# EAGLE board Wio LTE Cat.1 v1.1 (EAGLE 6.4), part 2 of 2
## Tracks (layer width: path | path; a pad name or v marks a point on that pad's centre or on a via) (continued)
N$49  (via drill 0.2 pad 0.41) (continued)
  VDD_3V3 0.305: v30.99,45.34 32,44.32 v33.91,44.32
N$50
  Top 0.127: U4.20 25.82,21.79 C28.1
N$51
  Bottom 0.127: U8.1 44.81,47.1 45.09,47.37 45.09,48.13 R81.1
N$52  (via drill 0.2 pad 0.41)
  Top 0.127: J11.2 8.27,40.66 v8,40.39
  Bottom 0.127: v8,40.39 7.87,40.51 R114.1 C57.1
N$53  (via drill 0.2 pad 0.41)
  Top 0.127: 17.78,6.42 v17.78,6.1 17.14,5.46 J10.3 | 17.78,6.42 D5.1 17.91,6.66 R17.1 | 17.78,6.42 17.78,6.6
  Bottom 0.127: v17.78,6.1 17.78,6.35 TP4.T
N$54  (via drill 0.2 pad 0.41)
  Top 0.127: J11.1 8.68,38.66 v8,37.97
  Bottom 0.127: R117.1 6.73,38.74 C62.1 v8,37.97
N$55  (via drill 0.2 pad 0.41)
  Top 0.127: 17.13,6.43 v17.13,6.09 16.5,5.46 J10.2 | 17.13,6.43 D3.1 17.02,6.66 R16.1 | 17.13,6.43 17.13,6.59 17.14,6.6
  Bottom 0.127: v17.13,6.09 17.13,6.37 TP3.T
N$56
  Top 0.127: R44.2 19.56,26.31 D17.-
N$57
  Bottom 0.127: U8.2 45.33,46.6 R96.1 R79.2
N$58
  Bottom 0.305: U8.3 R99.1
N$59
  Bottom 0.127: R25.2 11.81,12.19 12.95,11.05 20.32,11.05 24.13,7.24 25.53,7.24 26.29,6.48 28.51,6.48 28.89,6.1 D11.1 30.16,6.1 30.91,6.84 J2.P2B 38.59,6.84 40.64,8.89 40.64,12.06 40.01,12.7 J2.P2
  Bottom 0.152: C21.1 R25.2
N$60
  Bottom 0.127: 30.61,10.16 29.46,9.02 29.46,7.87 29.21,7.62 D10.1 28.89,7.62 28.51,8 24.64,8 21.21,11.43 13.84,11.43 13.34,11.94 R26.2 | 30.67,10.22 30.61,10.16 | 30.61,10.16 30.87,10.16 J2.P3B 37.75,10.44 38.96,11.66 J2.P3
  Bottom 0.152: C20.1 R26.2
N$61
  Bottom 0.305: C56.2 45.59,45.21 | 45.59,45.21 45.72,45.34 | 45.72,45.34 46.36,45.98 R99.2 | U8.4 45.2,45.6 45.42,45.38 | 45.42,45.38 45.59,45.21 | 45.42,45.38 45.68,45.38 45.72,45.34
N$62  (via drill 0.2 pad 0.41)
  Top 0.127: v41.53,9.27 v40.01,9.27 | v26.54,6.86 26.04,7.37 v26.04,8.64
  Bottom 0.127: v40.01,9.27 39.85,9.24 J2.P7B 30.87,9.24 29.84,8.22 29.84,7.49 29.21,6.86 D8.1 28.89,6.86 28.51,7.24 26.92,7.24 v26.54,6.86 | v41.53,9.27 41.53,5.33 38.96,2.77 J2.P7 | C19.1 14.1,12.19 14.48,11.81 21.21,11.81 24.38,8.64 v26.04,8.64
  Bottom 0.152: C19.1 R27.2 R23.2
N$63  (via drill 0.2 pad 0.41)
  Top 0.127: J12.3 7.6,28.69 v7.37,28.45
  Bottom 0.127: v7.37,28.45 7.24,28.58 C114.1 R118.1
N$64  (via drill 0.2 pad 0.41)
  Top 0.127: v7.37,27.3 8.26,27.3 8.87,26.69 J12.2
  Bottom 0.127: v7.37,27.3 7.24,27.43 R119.1 C64.1
N$65  (via drill 0.2 pad 0.41)
  Top 0.127: J12.1 8.46,24.69 8.13,25.02 v8.13,26.04
  Bottom 0.127: v8.13,26.04 7.75,26.04 7.24,26.55 R120.1 C115.1
N$66
  Top 0.127: Q9.3 35.43,4.95 R91.1
N$67  (via drill 0.25 pad 0.51)
  Top 0.127: J13.3 8.78,14.72 8.64,14.86 8.64,17.27 v8.26,17.65
  Bottom 0.127: C117.1 R121.1 v8.26,17.65
N$68
  Bottom 0.305: Q14.3 2.41,34.29 2.67,34.29 3.17,33.78 3.17,33.02 3.56,32.64 R103.1 3.56,32 Q13.1
N$69  (via drill 0.25 pad 0.51)
  Top 0.127: J13.2 8.75,12.72 8.38,13.08 8.38,15.49 v8.13,15.75
  Bottom 0.127: C116.1 7.88,15.5 v8.13,15.75 7.88,16 R122.1
N$70  (via drill 0.25 pad 0.51)
  Top 0.127: J13.1 8.46,10.72 7.87,11.3 v7.87,13.34
  Bottom 0.127: v7.87,13.34 v7.88,13.34 C126.1 R123.1
N$71
  Top 0.127: J15.3 36.43,26.69 35.81,27.3 35.81,29.59 34.54,30.86 C128.1 R129.1
N$72
  Top 0.127: U4.8 31.69,22.99 32,23.3 C42.2
N$73
  Top 0.127: J15.2 36.59,28.69 36.32,28.96 36.32,31.37 36.2,31.5 34.67,31.5 34.54,31.62 C127.1 R130.1
N$74
  Top 0.127: J15.1 37.26,30.69 36.7,31.24 36.7,32.26 36.32,32.64 34.67,32.64 34.54,32.77 C129.1 R131.1
N$75  (via drill 0.2 pad 0.41)
  Top 0.127: J16.3 42.24,12.72 v45.15,15.62
  Bottom 0.127: C131.1 45.21,15.62 v45.15,15.62 R124.1
N$76  (via drill 0.2 pad 0.41)
  Top 0.127: J16.2 43.35,14.72 v45.15,16.51
  Bottom 0.127: C130.1 v45.15,16.51 R127.1
N$77  (via drill 0.2 pad 0.41)
  Top 0.127: J16.1 44.53,16.72 45.15,17.34 v45.15,17.4
  Bottom 0.127: C132.1 v45.15,17.4 R128.1
N$78
  Top 0.127: U4.11 29.81,24.09 30.42,24.7 C26.2
N$79
  Top 0.127: U4.12 29.41,24.33 29.65,24.57 C26.1
N$80
  Top 0.127: U4.13 29.01,25.07 C27.2
N$81
  Top 0.127: U4.14 28.61,24.48 28.32,24.77 C27.1
N$82
  Bottom 0.127: Q3.3 8.51,9.27 7.24,10.54 Q2.1 5.59,10.54 5.08,11.05 5.08,12.95 R136.1
N$83
  Bottom 0.127: R135.1 C137.1 R137.2 4.44,5.21 Q3.1
N$85
  Top 0.127: U4.16 27.81,24.13 27.43,24.51 C36.1
N$87
  Top 0.127: Q6.1 31.37,33.78 R143.1 30.86,35.3 Q7.3
N$88
  Top 0.127: Q7.1 30.86,38.23 C143.1 | C143.1 R144.2 | C143.1 R142.1
N$89
  Top 0.254: U4.17 26.92,22.99 26.26,23.66 C29.1
N$90
  Top 0.203: C47.2 R53.1 | U4.29 29.41,18.21 C48.1
  Top 0.254: 29.41,18.22 C48.1 C47.2
N$93  (via drill 0.2 pad 0.41)
  Top 0.127: U4.21 26.28,21.39 v26.23,21.34
  VDD_3V3 0.127: v26.23,21.34 26.1,21.46 7.24,21.46 5.33,23.37 5.33,29.08 v5.84,29.59
  Bottom 0.127: v5.84,29.59 R42.2
N$94  (via drill 0.2 pad 0.41)
  Top 0.127: U4.22 26.45,20.99 26.29,20.83 v26.04,20.83 25.78,20.83 C44.1
  VDD_3V3 0.127: v26.04,20.83 25.65,21.21 7.11,21.21 5.08,23.24 5.08,30.48 v5.46,30.86
  Bottom 0.127: R41.2 v5.46,30.86
N$95  (via drill 0.2 pad 0.41)
  Top 0.127: U4.23 26.43,20.59 v26.16,20.32 26.04,20.32 25.91,20.19 C41.1
  VDD_3V3 0.127: v26.16,20.32 25.91,20.32 25.27,20.95 6.99,20.95 4.83,23.11 4.83,31.37 v5.08,31.62
  Bottom 0.127: v5.08,31.62 R40.2
N$96  (via drill 0.2 pad 0.41)
  Top 0.127: U4.24 26.79,20.19 v26.04,19.43 25.91,19.43 C40.1 25.53,18.92
  VDD_3V3 0.127: v26.04,19.43 24.77,20.7 6.86,20.7 4.57,22.99 4.57,32.38 v4.7,32.51
  Bottom 0.127: v4.7,32.51 R39.2
N$97
  Top 0.127: U4.32 32.41,19.59 R48.1
N$98
  Bottom 0.254: Q14.1 3.3,35.43 2.79,35.94 R102.1 R104.2 C91.1
N$99
  Top 0.127: U4.30 29.81,18.58 C46.1
N$100
  Bottom 0.305: Q15.1 3.56,19.94 R106.1 3.56,20.83 3.3,21.08 2.29,21.08 1.78,21.59 Q16.3
N$105
  Top 0.127: R91.2 34.16,3.51 D24.-
N$107
  Top 0.254: U4.19 25.69,22.19 C33.1
N$110
  Top 0.305: Q10.3 35.81,10.67 R93.1
N$111
  Top 0.127: R93.2 34.16,8.85 D25.-
N$113
  Bottom 0.305: R107.2 C93.1 R105.1 2.79,24.51 3.56,23.75 Q16.1 3.94,23.62
N$114
  Bottom 0.305: R109.2 C98.2 ANT1.D
N$115
  Bottom 0.305: R110.2 C100.2 | C100.2 25.45,52.07 L1.1 | C100.2 ANT2.D
N$118
  Bottom 0.305: L1.2 26.4,52.98 R111.1
N$120
  Top 0.127: R70.2 R71.1 36,19.65 C80.2
N$121
  Top 0.127: R72.1 R73.2 35.37,19.65 C80.1
N$123
  Top 0.127: J3.1 31.1,2.79 31.5,2.79 32.13,3.43 32.13,4.57 32.96,5.4 32.96,12.37 32.37,12.95 31.5,12.95 31.11,13.34 R82.2
N$129
  Top 0.127: 36.29,1.14 K3.4 36.58,1.43 36.58,1.91 36.57,1.91 R29.1
N$130
  Top 0.127: R30.1 7.11,5.33 7.87,6.1 9.65,6.1 10.46,5.28 K4.4
N$132
  Top 0.127: R78.2 21.59,5.78 D18.1 21.66,3.74 21.97,3.43 23.68,3.43 J3.6
N$134
  Top 0.127: J3.2 31.18,5.08 32.26,5.08 32.64,5.46 32.64,11.94 32,12.57 31.24,12.57 30.35,13.46 R75.2
NET_MODE  (via drill 0.2 pad 0.41)
  Top 0.127: R94.2 34.16,13.08 v34.04,12.95 Q10.1
  Bottom 0.127: U1.5 31.75,16.51 31.75,16 32.26,15.49 33.02,15.49 33.4,15.11 33.4,13.72 34.04,13.08 v34.04,12.95
NET_STATUS  (via drill 0.2 pad 0.41)
  Top 0.127: R92.2 34.16,7.24 Q9.1 33.4,6.99 v33.4,12.64
  Bottom 0.127: v33.4,12.64 33.4,13.21 33.02,13.59 33.02,14.99 32.77,15.24 31.24,15.24 30.35,16.13 30.35,16.61 U1.6
NRST  (via drill 0.2 pad 0.41)
  Top 0.127: 33.91,2.35 33.12,2.35 D14.- | 33.91,2.35 37.27,2.35 v38.35,3.43 | U3.7 21.7,42.05 21.34,42.42 20.57,42.42 19.81,43.18 v19.81,44.32 C23.1 | D27.1 33.91,2.35
  Top 0.305: K3.2 38.41,3.48 v38.35,3.43
  VDD_3V3 0.203: v38.35,3.43 19.18,3.43 18.54,4.06 18.54,6.1 16.89,7.75 14.1,7.75 13.34,8.51 9.02,8.51 5.97,11.56 5.97,20.45 3.68,22.73 3.68,32.89 1.91,34.67 v1.91,38.73 1.91,45.74 3.16,46.99 18.16,46.99 19.81,45.34 v19.81,44.32
  Bottom 0.305: v1.91,38.73 J4.5 | J4.5
OE
  Top 0.127: R89.1 R125.1 | R125.1 17.65,19.56 17.78,19.68 18.67,19.68 18.8,19.82 U9.10 | R125.1 R126.2
OSC32_IN
  Top 0.127: U3.3 23.7,42.12 24,42.42 25.27,42.42 25.78,42.93 C10.1 25.72,43.43 25.34,43.81 25.34,44.51 26.02,45.2 X1.1
OSC32_OUT
  Top 0.127: U3.4 23.2,42.38 23.5,42.67 24.38,42.67 24.64,42.93 C11.1 25.08,43.88 25.08,44.51 24.4,45.2 X1.2
OSC_IN
  Top 0.127: U3.5 22.7,42.64 23.37,43.31 23.37,43.76 X3.1
OSC_OUT
  Top 0.127: U3.6 22.2,42.18 21.21,43.18 21.21,43.63 X3.3
PWRKEY  (via drill 0.2 pad 0.41)
  Top 0.127: K4.2 6.88,1.38 6.1,2.16 D26.1 | 6.06,5.23 D26.1 | v6.6,18.67 7.11,18.16 7.11,14.48 6.86,14.22 6.86,12.95 5.59,11.68 5.59,5.46 5.78,5.26 D26.1
  Bottom 0.127: U1.21 9.18,25.18 8.51,24.51 6.6,24.51 6.29,24.19 6.29,21.59 7.11,20.77 R85.1 6.99,20.2 6.22,19.43 R37.2 6.1,19.18 v6.6,18.67
PWRKEY_MODULE  (via drill 0.2 pad 0.41)
  Top 0.127: v6.99,24.13 6.99,34.67 8.64,36.32 13.72,36.32 14.23,35.81 U3.24
  Bottom 0.127: v6.99,24.13 7.18,23.94 Q1.1 8,23.5 R38.2
RESET_MODULE
  Top 0.127: U3.11 19.7,34.5 16,30.8 16,27.56 16.2,27.36 U9.15
RESET_N  (via drill 0.2 pad 0.41)
  Top 0.127: U9.6 16.2,21.79 v16.26,21.84
  VDD_3V3 0.127: v16.26,21.84 16.13,21.72 13.21,21.72 v11.43,23.5
  Bottom 0.127: v11.43,23.5 11.43,23.62 11.17,23.88 U1.20
RGB_POWR  (via drill 0.2 pad 0.41)
  Top 0.127: U3.41 21.2,30.48 22.73,32 v22.73,35.81
  Bottom 0.127: R8.2 8.13,37.21 8.38,37.47 11.56,37.47 13.08,35.94 17.02,35.94 17.78,35.18 20.7,35.18 21.34,35.81 v22.73,35.81
RI_MODULE  (via drill 0.2 pad 0.41)
  Top 0.127: U9.1 12.95,24.38 v13.84,25.27
  Bottom 0.127: v13.84,25.27 15.88,25.27 16.64,26.04 16.64,27.84 18.01,29.21 20.57,29.21 24.13,32.77 26.16,32.77 26.54,33.15 26.54,34.54 26.92,34.92 36.77,34.92 37.42,35.58 U1.62
RX_LED
  Top 0.127: U3.34 17.7,28.4 18.41,27.69 18.42,27.69 R44.1
RXD_MODULE  (via drill 0.2 pad 0.41)
  Top 0.127: U9.5 15.55,21.77 16.38,22.61 v17.4,22.61
  Bottom 0.127: v17.4,22.61 17.4,24.77 17.78,25.15 35.18,25.15 36.07,26.04 36.07,27.18 36.67,27.78 U1.68
SD_CLK
  Bottom 0.127: J2.T5 37.91,15.23 38.69,16 41.4,16 41.91,16.51 D20.1 42.09,17.2 C18.1 R64.2 R60.1
SD_CMD
  Bottom 0.127: J2.T3 36.86,1.49 36.45,1.91 36.45,2.67 35.69,3.43 28.32,3.43 27.11,4.64 26.23,4.64 26.04,4.83 D22.1 25.97,5.08 C17.1 R58.1 R63.2
SD_DATA0
  Bottom 0.102: 38.92,16.51 38.86,16.51 37.47,15.11 36.32,15.11 35.81,14.6
  Bottom 0.127: R61.1 R65.2 C60.1 40.13,16.58 D19.1 38.92,16.51 | J2.T7 35.81,14.6
SD_POWR  (via drill 0.2 pad 0.41)
  Top 0.127: U3.50 24.97,32.31 24,33.27 v24,34.16
  VDD_3V3 0.127: v4.83,36.45 6.86,34.42 20.32,34.42 20.83,33.91 23.75,33.91 v24,34.16
  Bottom 0.127: v4.83,36.45 4.7,36.58 R102.2
SDIO_CK  (via drill 0.2 pad 0.41)
  Top 0.127: U3.53 27.51,33.81 27.88,33.44 v27.88,29.15
  Bottom 0.127: v27.88,29.15 27.94,29.21 35.05,29.21 36.83,30.99 40.39,30.99 41.4,29.97 42.42,29.97 43.81,28.57 43.81,20.32 R60.2
SDIO_CMD  (via drill 0.2 pad 0.41)
  Top 0.127: U3.54 25.8,34.31 v25.78,34.29
  VDD_3V3 0.127: v25.78,34.29 25.4,33.91 25.4,33.02 26.04,32.38 26.04,28.7 27.18,27.56 27.18,20.04 27.54,19.68 28.77,19.68 29.21,19.24 29.21,18.34 28.71,17.84 26.86,17.84 26.67,17.65 25.02,17.65 24.26,16.89 24.26,10.03 22.8,8.57 v22.23,8.57
  Bottom 0.127: v22.23,8.57 24.38,6.41 R58.2
SDIO_D0  (via drill 0.2 pad 0.41)
  Top 0.127: U3.39 20.2,29.16 21.04,28.32 v21.14,28.32
  Bottom 0.127: R61.2 41.4,20.07 43.05,20.07 43.56,20.57 43.56,28.44 42.28,29.72 36.58,29.72 35.24,28.38 21.21,28.38 v21.14,28.32
SDIO_D1  (via drill 0.2 pad 0.41)
  Top 0.127: U3.40 20.7,30.61 v21.21,31.11
  VDD_3V3 0.127: v23.11,11.3 23.75,11.94 23.75,17.14 24.77,18.16 26.42,18.16 26.61,18.35 28.44,18.35 28.7,18.61 28.7,18.99 28.51,19.18 27.18,19.18 26.67,19.68 26.67,24.38 21.21,29.84 v21.21,31.11
  Bottom 0.127: R57.2 v23.12,11.3 v23.11,11.3
SDIO_D2  (via drill 0.2 pad 0.41)
  Top 0.127: U3.51 25.48,32.81 v25.02,33.27
  VDD_3V3 0.127: v21.72,8.38 21.72,8.64 22.23,9.14 22.99,9.14 24,10.16 24,17.02 24.89,17.91 26.54,17.91 26.73,18.1 28.59,18.1 28.96,18.47 28.96,19.11 28.64,19.43 27.38,19.43 26.92,19.89 26.92,27.43 25.78,28.57 25.78,32.26 25.02,33.02 v25.02,33.27
  Bottom 0.127: R5.2 24.38,1.02 24.26,0.89 23.11,0.89 21.46,2.54 21.46,8.13 v21.72,8.38
SDIO_D3  (via drill 0.2 pad 0.41)
  Top 0.127: U3.52 25.82,33.31 v25.78,33.27
  VDD_3V3 0.127: v25.78,33.27 26.29,32.77 26.29,28.83 27.43,27.69 27.43,20.19 27.69,19.94 28.96,19.94 29.46,19.43 29.46,18.22 28.83,17.59 27.05,17.59 26.86,17.4 25.15,17.4 24.51,16.76 24.51,9.91 22.61,8 v22.23,8
  Bottom 0.127: R24.2 23.12,3.17 22.86,3.43 22.86,4.32 21.84,5.33 21.84,7.62 v22.23,8
SPK_L
  Top 0.203: C28.2 24.26,21.46 23.75,20.95 23.75,18.67 arc90 24,18.41 24.45,18.41 arc-90 24.7,18.16 arc-90 24.45,17.91 24,17.91 arc90 23.75,17.65 arc90 24,17.4 24.45,17.4 arc-90 24.7,17.14 arc-90 24.45,16.89 24,16.89 arc90 23.75,16.51 23.75,15.05 23.88,14.92 24.13,14.92 C88.2 C87.1 C96.1 26.73,15.05 26.8,15.11 D9.1 27.4,15.3 R83.1
SPK_R
  Top 0.203: C29.2 25.11,24.86 24.51,24.26 24.51,23.37 23.37,22.23 23.37,14.92 23.69,14.61 24,14.61 24.13,14.48 C86.2 C89.2 C97.2 26.74,14.48 D13.1 27.27,14.42 R84.1
STATUS  (via drill 0.2 pad 0.41)
  Top 0.127: v21.27,34.29 18.7,31.72 U3.36 18.7,28.79 19.18,28.32 20.45,28.32 R101.1
  Bottom 0.127: v21.27,34.29 22.04,35.05 25.02,35.05 25.78,35.81 35.89,35.81 36.96,36.88 U1.61
TX_LED
  Top 0.127: U3.35 18.2,28.66 18.8,28.07 19.94,28.07 R43.1
TXD_MODULE  (via drill 0.2 pad 0.41)
  Top 0.127: U9.4 14.9,22.14 v14.99,22.23
  Bottom 0.127: v14.99,22.23 16.38,22.23 17.14,22.99 17.14,25.15 17.4,25.4 34.92,25.4 35.69,26.16 35.69,28.07 36.7,29.08 U1.67
USART1_RX
  Top 0.127: R131.2 33.02,36.07 32.13,36.96 28.45,36.96 28.3,36.81 U3.59
USART1_TX
  Top 0.127: U3.58 28.18,36.31 28.57,36.7 31.88,36.7 32.26,36.32 32.26,32.38 32.64,32 R130.2
USART2_RX
  Top 0.127: U3.17 17.71,39.31 18.16,38.86 18.16,33.72 15.49,31.05 15.49,27.81 14.9,27.22 U9.17
USART2_TX
  Top 0.127: U3.16 17.2,40.2 18.41,38.99 18.41,33.59 15.75,30.92 15.75,27.43 15.55,27.23 U9.16
USB_BOOT
  Bottom 0.127: R86.1 R87.2 8.63,20.83 9.09,21.28 U1.115
USB_DM
  Bottom 0.203: R9.2 TP14.T
USB_DP
  Bottom 0.203: R10.2 41.91,26.04 TP15.T
USB_FS_DM
  Top 0.127: U3.44 22.7,29.11 22.86,28.96 22.86,24.89 21.59,23.62 21.59,9.91 20.7,9.02 17.65,9.02 17.34,8.7 17.34,8.38 17.08,8.13 R16.2
USB_FS_DP
  Top 0.127: U3.45 23.2,29.05 23.11,28.96 23.11,24.77 21.84,23.5 21.84,9.78 20.83,8.76 17.78,8.76 17.59,8.57 17.59,8.38 17.84,8.13 R17.2
USB_FS_VBUS
  Top 0.254: U3.42 21.7,27.7 R95.2
USB_VBUS
  Bottom 0.406: U1.71 41.52,23.88 TP13.T
USIM_CLK
  Bottom 0.127: U1.16 14.13,15.15 R26.1
USIM_DATA
  Bottom 0.127: U1.15 15.43,14.92 R27.1
USIM_GND  (via drill 0.2 pad 0.41)
  Top 0.127: v42.04,6.35 v40.01,6.35 | v32.19,5.64 32.19,11.75 31.75,12.19 30.99,12.19 30.23,12.95 v23.37,12.95
  Bottom 0.127: 32,5.64 J2.P5B v32.19,5.64 39.3,5.64 v40.01,6.35 | J2.P5 41.06,4.49 42.04,5.46 v42.04,6.35 | 21.97,13.59 C59.1 C58.2 | U1.10 21.93,13.63 21.97,13.59 | 21.97,13.59 22.73,13.59 v23.37,12.95
USIM_RST
  Bottom 0.203: U1.17 12.83,16.13 11.81,15.11 R25.1
USIM_VDD  (via drill 0.2 pad 0.41)
  Top 0.127: v26.92,5.71 26.92,7.24 26.42,7.75 26.42,8.89 v26.16,9.14
  Bottom 0.127: J2.P1 41.06,6.72 38.78,4.44 J2.P1B 30.86,4.44 29.97,5.33 D12.1 28.89,5.33 28.51,5.71 v26.92,5.71 | R23.1 C58.1 | C58.1 17.15,12.32 17.14,12.32 17.14,15.24 16.73,15.65 U1.14 | C58.1 17.91,12.06 21.33,12.06 21.34,12.06 24.26,9.14 v26.16,9.14
VBAT  (via drill 0.2 pad 0.41)
  Top 0.305: v45.59,43.05 v42.16,43.05
  Bottom 0.305: R97.1 v45.59,43.05 | C55.1 42.83,43.34 42.55,43.05 v42.16,43.05
  Bottom 0.381: C107.2 41.15,40.83
  Bottom 0.508: TP5.T 42.93,37.91 C77.+
  Bottom 0.61: C113.+ 42.93,41.15 42.04,40.26
  pour Bottom (isolate 0.127, no thermals): 42.55,37.4 37.34,37.4 36.96,37.79 36.96,39.47 37.24,39.75 38.94,39.75 39.12,39.57 39.12,39.24 39.62,38.73 42.55,38.73
  pour Bottom (isolate 0.127, no thermals): 41.78,38.73 41.78,36.99 42.07,36.7 43.79,36.7 44.07,36.99 44.07,37.85 43.18,38.73
  pour Bottom (isolate 0.127, no thermals): 41.91,42.04 37,42.04 36.77,41.81 36.77,40.67 37.17,40.26 38.86,40.26 39.24,40.64 41.91,40.64
  pour Bottom (isolate 0.254, rank 2, no thermals): 42.67,44.83 41.91,44.83 41.02,43.94 41.02,43.31 41.78,42.55 41.78,39.12 42.42,38.35 43.43,38.35 43.81,38.73 43.81,42.29 43.18,42.93 43.18,44.32
VDD_1V8  (via drill 0.2 pad 0.41)
  Top 0.254: R55.2 R54.2 v33.2,22.54 33.34,22.54 | C65.2 | C65.2 v14.8,18.22 | U9.2 13.6,18.91 13.97,18.54 C65.2 | R53.2 v27.94,16.95 | R89.2 v16.89,18.16
  Top 0.305: R52.2 29.46,25.91 v29.59,25.78 | TP8.T 32.89,26.04 v32.64,25.78 | v28.45,32.38 28.96,32.38 Q6.2 30.1,33.53 R143.2
  Top 0.406: U11.2 C120.2 34.04,26.42 TP8.T
  VDD_3V3 0.254: 15.05,18.67 14.73,18.67 | 14.73,18.67 14.54,18.67 | v14.8,18.22 14.8,18.41 | 14.8,18.41 14.8,18.61 14.73,18.67 | 14.54,18.67 14.8,18.41 | 15.05,18.67 14.8,18.41 | v32.64,25.78 33.2,25.22 v33.2,22.54 33.2,18.47 31.69,16.95 v27.94,16.95 | v22.86,12.45 22.86,16.51 20.7,18.67 17.14,18.67 | 15.05,18.67 16.64,18.67 | 16.64,18.67 16.89,18.67 | 16.89,18.67 17.14,18.67 | 14.54,18.67 14.41,18.67 14.16,18.92 8.38,18.92 v8.26,18.8 | 16.89,18.67 16.89,18.41 | 16.89,18.41 v16.89,18.16 | 16.64,18.67 16.89,18.41 | 17.14,18.67 16.89,18.41
  VDD_3V3 0.305: v32.64,25.78 v29.59,25.78 29.59,28.32 28.19,29.72 28.19,32.13 v28.45,32.38
  Bottom 0.254: R85.2 7.11,19.05 7.37,18.8 v8.26,18.8 | v22.86,12.45 23.62,12.45 26.16,14.99 27.18,14.99 27.94,15.75 v27.94,16.95
VDD_1V8_I2C  (via drill 0.2 pad 0.41)
  Top 0.127: R50.2 R51.2 27.18,17.02 28.19,16 v28.19,14.86 | v31.11,27.3 31.08,27.34 C142.1 31.08,30.39 Q6.3
  VDD_3V3 0.127: v28.19,14.86 28.96,14.1 30.61,14.1 34.29,17.78 34.29,24.77 31.75,27.3 v31.11,27.3
  Bottom 0.127: R141.2 v28.19,14.86
VDD_3V3  (via drill 0.2 pad 0.41)
  Top 0.203: R101.2 21.08,26.67 21.72,26.04 21.72,24.89 v21.59,24.77 21.54,24.81 D6.+
  Top 0.254: U3.19 13.61,38.31 | 13.61,38.31 C30.2 C31.2 12.83,38.61 v12.7,38.73 | U3.32 14.22,31.81 v14.29,31.88 13.91,31.5 C32.2 C68.2 | U9.19 13.6,27.82 C76.2 13.65,27.94 12.89,28.7 R100.2 | U3.48 24.7,27.75 C70.2 C71.2 | D6.+ D17.+ | 13.61,38.31 13.61,38.46 v13.34,38.73 | R31.1 33.53,3.05 33.78,2.79 v35.05,2.79
  Top 0.305: R36.2 C75.2 C66.2 R35.2 28.07,39.88 27.5,39.31 U3.64 | C38.2 C39.2 26.54,42.55 25.31,41.31 U3.1 | D24.+ 35.05,3.43 v35.05,2.79 | R74.1 20.83,7.62 20.83,7.75 20.57,8 v19.94,8 | v25.97,27.69 C71.2 | v36.45,18.16 34.54,18.16 33.78,17.4 R145.2 | D25.+ v36.07,8.76 | L12.1 17.02,45.21 v16.26,44.45
  Top 0.381: R77.2 v12.57,33.78 | C76.2 14.1,27.94 14.48,28.32 v14.48,28.57
  Top 0.406: C38.2 v27.3,42.93 | R36.2 28.07,42.16 v27.69,42.55 | R45.2 v29.08,46.23 | R77.2 R56.2
  VDD_3V3 0.305: v36.45,18.16 37.72,18.16 v38.1,18.54
  Bottom 0.305: v0.95,47.82 J4.1 4,47.81 5.21,46.61 5.21,44.64 4.38,43.81 R15.2 R18.2 | R103.2 v2.79,31.75 | v3.17,30.48 Q13.2 | R106.2 v2.41,20.45 | v3.17,17.53 Q15.2 | TP12.T 40.01,20.95 39.5,20.45 39.5,19.43 38.61,18.54 v38.1,18.54 | R113.2 v6.35,42.04 | R139.2 4.96,38.61 4.45,39.12 4.45,41.02 v4.32,41.15 Q4.2 | v19.94,8 v12.06,8
  Bottom 0.406: v3.56,13.08 3.49,13.14 R11.2 3.49,13.78 4.07,14.35 R136.2 5.21,14.35 6.48,13.08 Q2.2
  other vias: 35.31,46.23 35.31,45.72
  pour Top (isolate 0.127, no thermals): 34.29,44.58 35.56,44.58 35.56,47.88 34.29,47.88
  pour VDD_3V3 (isolate 0.203, rank 6): 0.64,0.64 46.99,0.64 46.99,49.13 46.59,49.53 40.89,49.66 39.62,48.39 0.64,48.26
VDD_3V3_B  (via drill 0.2 pad 0.41)
  Top 0.406: v5.84,28.38 5.78,28.38 5.33,27.94 v5.33,17.65 | R132.2 34.54,38.73 34.16,38.35 v32.26,38.35 | R129.2 v31.62,30.99
  VDD_3V3 0.406: 31.24,30.61 31.24,30.1 33.02,28.32 38.1,28.32 40.01,26.42 v40.01,15.37 | 31.24,30.61 31.24,30.99 | 31.24,30.99 31.24,31.37 | 31.24,31.37 31.24,37.34 v32.26,38.35 | 31.24,30.99 v31.62,30.99 | 31.24,31.37 v31.62,30.99 | 31.24,30.61 v31.62,30.99 | v5.33,17.65 5.46,17.53 5.46,11.18 9.14,7.49 v10.03,7.49 | v5.84,28.38 5.84,28.32 6.22,27.94 9.14,27.94 14.1,32.89 22.99,32.89 v24.64,31.24
  Bottom 0.406: R124.2 43.69,15.62 43.43,15.37 v40.01,15.37 | R118.2 v5.84,28.39 v5.84,28.38 | R121.2 v5.33,17.65 | Q2.3 9.11,10.83 C136.1 v10.03,7.49 | v31.62,30.99 30.73,31.88 25.27,31.88 v24.64,31.24
VDD_3V3_RGB
  Bottom 0.406: Q4.3 C140.1 6,42.45 6.35,42.8 R6.1
VDD_3V3_SD  (via drill 0.2 pad 0.41)
  Top 0.203: C16.2 39.24,2.48 v39.24,3.68
  Top 0.305: v22.35,5.59 22.35,4.95 | 22.35,4.95 v22.35,3.94 | 22.35,4.95 25.65,4.95 26.29,5.59 26.29,6.22 25.53,6.99 25.53,9.27 v26.04,9.78
  Top 0.406: v40.89,18.92 v43.43,18.92 | v7.62,25.65 7.49,25.53 7.49,14.22 7.24,13.97 7.24,11.05 9.27,9.02 v11.68,9.02
  VDD_3V3 0.406: v11.68,9.02 13.72,9.02 14.48,8.26 17.14,8.26 21.46,3.94 v22.35,3.94 38.99,3.94 v39.24,3.68 40.26,2.67 42.04,2.67 43.31,3.94 43.31,18.8 v43.43,18.92
  Bottom 0.203: J2.T4 37.91,2.35 v39.24,3.68
  Bottom 0.254: R62.1 24.38,2.79 24.26,2.67
  Bottom 0.305: 24.26,2.67 22.99,2.67 | 22.99,2.67 22.73,2.67 | 22.73,2.67 22.35,3.05 v22.35,3.94 | R76.1 23.12,1.4 22.73,1.78 22.73,2.41 | 22.73,2.41 22.73,2.67 | 22.73,2.41 22.99,2.67 | R63.1 22.61,5.84 v22.35,5.59 | R80.1 24.38,10.16 24.77,9.78 v26.04,9.78
  Bottom 0.406: C79.1 3.84,28.03 | 3.84,28.03 3.05,28.83 3.05,29.59 Q13.3 | R65.1 v40.9,18.92 v40.89,18.92 | 3.84,28.03 4.19,27.69 4.19,26.67 5.21,25.65 v7.62,25.65 | R64.1 v43.43,18.92
VDD_ANT  (via drill 0.2 pad 0.41)
  VDD_3V3 0.305: v25.78,51.18 25.78,49.28 24.13,47.62 3.17,47.62 1.27,45.72 1.27,18.29 v2.16,17.4
  Bottom 0.305: R111.2 C101.2 v25.78,51.18 | C92.1 2.16,16.54 v2.16,17.4 Q15.3 2.03,18.41
VDD_EXT  (via drill 0.2 pad 0.41)
  Top 0.127: R125.2 v17.65,18.16
  VDD_3V3 0.127: v17.65,18.16 17.27,17.78 14.73,17.78 13.97,18.54 8.83,18.54 v8.76,18.48
  Bottom 0.127: R86.2 8.51,19.43 8.76,19.18 v8.76,18.48 | R141.1 28.57,13.71 28.7,13.84 28.7,15.49 28.93,15.72 U1.7 28.93,17.23 28.32,17.84 17.97,17.84 v17.65,18.16
VDDA/VREF+
  Top 0.305: U3.13 18.7,42.51 18.54,42.67 C118.2 C119.2 | C119.2 17.49,44.07 C139.1 | C119.2 18.54,45.08 L12.2
VSYS  (via drill 0.2 pad 0.41, 0.25 pad 0.51)
  Top 0.203: U5.1 16.9,12.97 16.51,12.57 U5.15
  Top 0.254: v14.73,15.49 13.93,16.3 D16.+
  Top 0.279: U5.1 18.4,12.97 v18.41,12.95
  Top 0.305: R90.2 v29.21,45.34 | U6.7 30.74,43.18 30.61,43.05 | U6.8 30.75,42.68 30.73,42.67 | v43.18,49.15 43.56,49.53 46.61,49.53 46.99,49.15 46.99,48.39 v46.74,48.13
  Top 0.406: v31.88,30.35 32,30.23 C2.2 33.78,29.97 U11.3
  Top 0.61: C24.1 18.83,17.49 19.67,16.65 L6.2
  VDD_3V3 0.406: v18.41,12.95 18.29,12.83 v18.29,12.51 17.97,12.51 17.91,12.57 | v31.88,30.35 33.15,30.35
  VDD_3V3 0.508: 17.91,12.57 17.91,13.34 | 17.97,12.51 17.72,12.51 17.65,12.57 17.65,13.34 17.78,13.46
  VDD_3V3 1.016: 17.91,13.34 18.41,13.84 19.43,13.84 | 19.43,13.84 20.19,13.84 | 20.19,13.84 20.7,13.84 21.34,13.21 | 21.34,13.21 21.34,13.97 | 21.34,13.97 19.94,15.37 | 19.94,15.37 19.56,15.75 19.56,17.53 | 19.94,15.37 19.94,14.35 | 19.94,14.35 19.94,14.1 20.19,13.84 | 19.43,13.84 19.94,14.35 | 41.78,28.83 41.78,15.75 39.88,13.84 32.13,13.84 30.35,12.06 30.35,9.14 28.96,7.75 25.02,7.75 24,6.73 22.1,6.73 20.83,8 20.83,9.14 21.59,9.91 21.59,12.95 21.34,13.21 | 41.78,28.83 41.78,29.59 | 21.34,13.97 21.34,15.37 | 41.78,28.83 42.42,29.46 | 41.78,28.07 41.78,28.45 40.51,29.72
  Bottom 0.305: C13.2 42.83,48.8 v43.18,49.15
  Bottom 0.406: R79.1 46.36,47.75 v46.74,48.13
  other vias: 42.8,47.5 42.16,47.5 42.16,48.13 29.34,43.18 29.34,42.67 19.68,18.22 19.18,18.22
  pour VDD_3V3 (isolate 0.203): 28.83,42.93 32.77,38.99 32.77,29.97 32.77,29.97 33.65,29.1 43.32,29.09 44.32,30.09 44.32,46.48 42.28,48.49 41.31,48.47 38.73,45.72 29.01,45.72 28.83,45.54
  pour Bottom (isolate 0.254, rank 2, no thermals): 42.67,46.86 42.29,46.86 41.91,47.24 41.91,48.51 42.04,48.64 42.93,48.64 43.05,48.51 43.05,46.99 42.93,46.86
  pour Top (isolate 0.254, no thermals): 28.57,43.43 30.48,43.43 30.61,43.31 30.86,43.31 30.99,43.18 30.99,42.04 30.86,41.91 28.83,41.91 28.19,42.55 28.19,43.31 28.32,43.43
  pour Top (isolate 0.254, no thermals): 17.78,13.08 18.54,13.08 18.67,12.95 18.67,12.45 18.54,12.32 17.78,12.32 17.65,12.45 17.65,12.95
  pour Top (isolate 0.254, no thermals): 20.45,16.13 19.43,16.13 19.18,16.38 19.18,16.76 18.8,17.14 18.16,17.14 17.91,17.4 17.91,18.16 18.03,18.29 18.8,18.29 18.92,18.41 18.92,19.05 19.05,19.18 19.81,19.18 19.94,19.05 19.94,18.29 20.7,17.53 20.7,16.38
  pour VDD_3V3 (isolate 0.254, no thermals): 18.41,18.41 20.21,18.41 22.1,16.53 22.1,14.48 21.72,14.1 20.95,14.1 19.18,15.88 15.37,15.88 14.86,15.37 14.73,15.37 14.61,15.49 14.61,17.04 14.96,17.4 17.4,17.4
W_DISABLE
  Top 0.127: U3.10 20.2,34.62 16.26,30.67 16.26,27.81 16.84,27.23 U9.14
W_DISABLE_MODULE  (via drill 0.2 pad 0.41)
  Top 0.127: U9.7 16.85,22.06 v16.89,22.1
  Bottom 0.127: U1.4 32.83,17.21 31.94,18.1 20.51,18.1 19.94,18.67 19.94,19.68 19.68,19.94 18.54,19.94 18.03,20.45 18.03,21.59 17.53,22.1 v16.89,22.1
WAKEUP_IN
  Top 0.127: U3.8 21.2,34.86 16.76,30.42 16.76,28.57 18.14,27.2 U9.12
WAKEUP_IN_MODULE  (via drill 0.2 pad 0.41)
  Top 0.127: U9.9 18.15,21.71 v18.67,22.23
  Bottom 0.127: U1.1 36.73,17.25 35.81,18.16 32.64,18.16 32.13,18.67 32.13,19.56 31.81,19.88 20.51,19.88 19.94,20.45 19.94,21.72 19.56,22.23 v18.67,22.23

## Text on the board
tNames: Wio LTE Cat.1 | GND | v1.1 10/11/2017 | SCL | 3V3 | RGB | SDA | D38 | I2C | 3V3 | D38 | D39 | GND | GND | 3V3 | RX | TX | D20 | 3V3 | UART | GND | D19 | D20 | GND | 3V3 | A4 | A5 | A6 | A4 | A7 | 3V3 | A6 | GND | PWR | RST | - | + | C:/Users/Dwin/Desktop/satellite-gps-icon-86608.bmp | RST
bNames: Main | BOOT0
dxf: F | F | F | F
